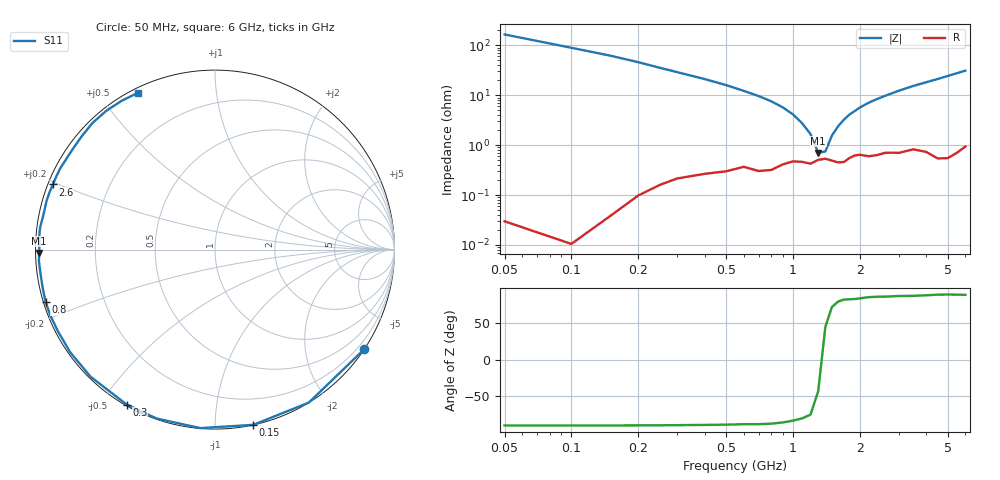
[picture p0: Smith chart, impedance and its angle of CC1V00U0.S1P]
! Infineon Technologies  Discrete & RF Semiconductors
! BBY57-02W
! Si Tuning Diode in SCD-80
! VR = 1 V
! S-Parameters:  June  2000
# GHz  S  MA  R  50
!  f  S11
! GHz  MAG  ANG
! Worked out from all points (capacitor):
!   34 points, 50 MHz to 6 GHz, reference 50 ohm
!   read as one part to ground: C = 17.7 pF near 50 MHz
!   lowest |Z| = 699 mohm at 1.3 GHz (marker M1)
!   series resonance near 1.348 GHz, so ESL is about 790 pH
!   S11 on the Smith chart (normalised r, x): 50 MHz: 0.00, -3.30; 150 MHz: 0.00, -1.24; 300 MHz: 0.00, -0.58; 800 MHz: 0.01, -0.15; 2.6 GHz: 0.01, +0.19; 6 GHz: 0.02, +0.62
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0.05  0.9999 -33.7
0.1  0.9999 -58.5
0.15  0.9994 -77.7
0.2  0.9979 -94.7
0.25  0.9958 -109.1
0.3  0.9936 -119.7
0.4  0.991 -134.3
0.5  0.9892 -144.7
0.6  0.9862 -152.5
0.7  0.9884 -158.2
0.8  0.9876 -162.9
0.9  0.9839 -167.0
1  0.9814 -170.6
1.1  0.9817 -173.8
1.2  0.9832 -176.3
1.3  0.9799 -178.9
1.6  0.9822 174.6
1.8  0.9783 170.7
2  0.975 167.2
2.4  0.9757 160.9
2.6  0.9734 158.1
3  0.974 152.4
3.5  0.9703 145.8
4  0.9746 139.9
4.5  0.9818 134.1
5  0.9824 128.0
5.5  0.9786 122.1
6  0.9734 116.2
